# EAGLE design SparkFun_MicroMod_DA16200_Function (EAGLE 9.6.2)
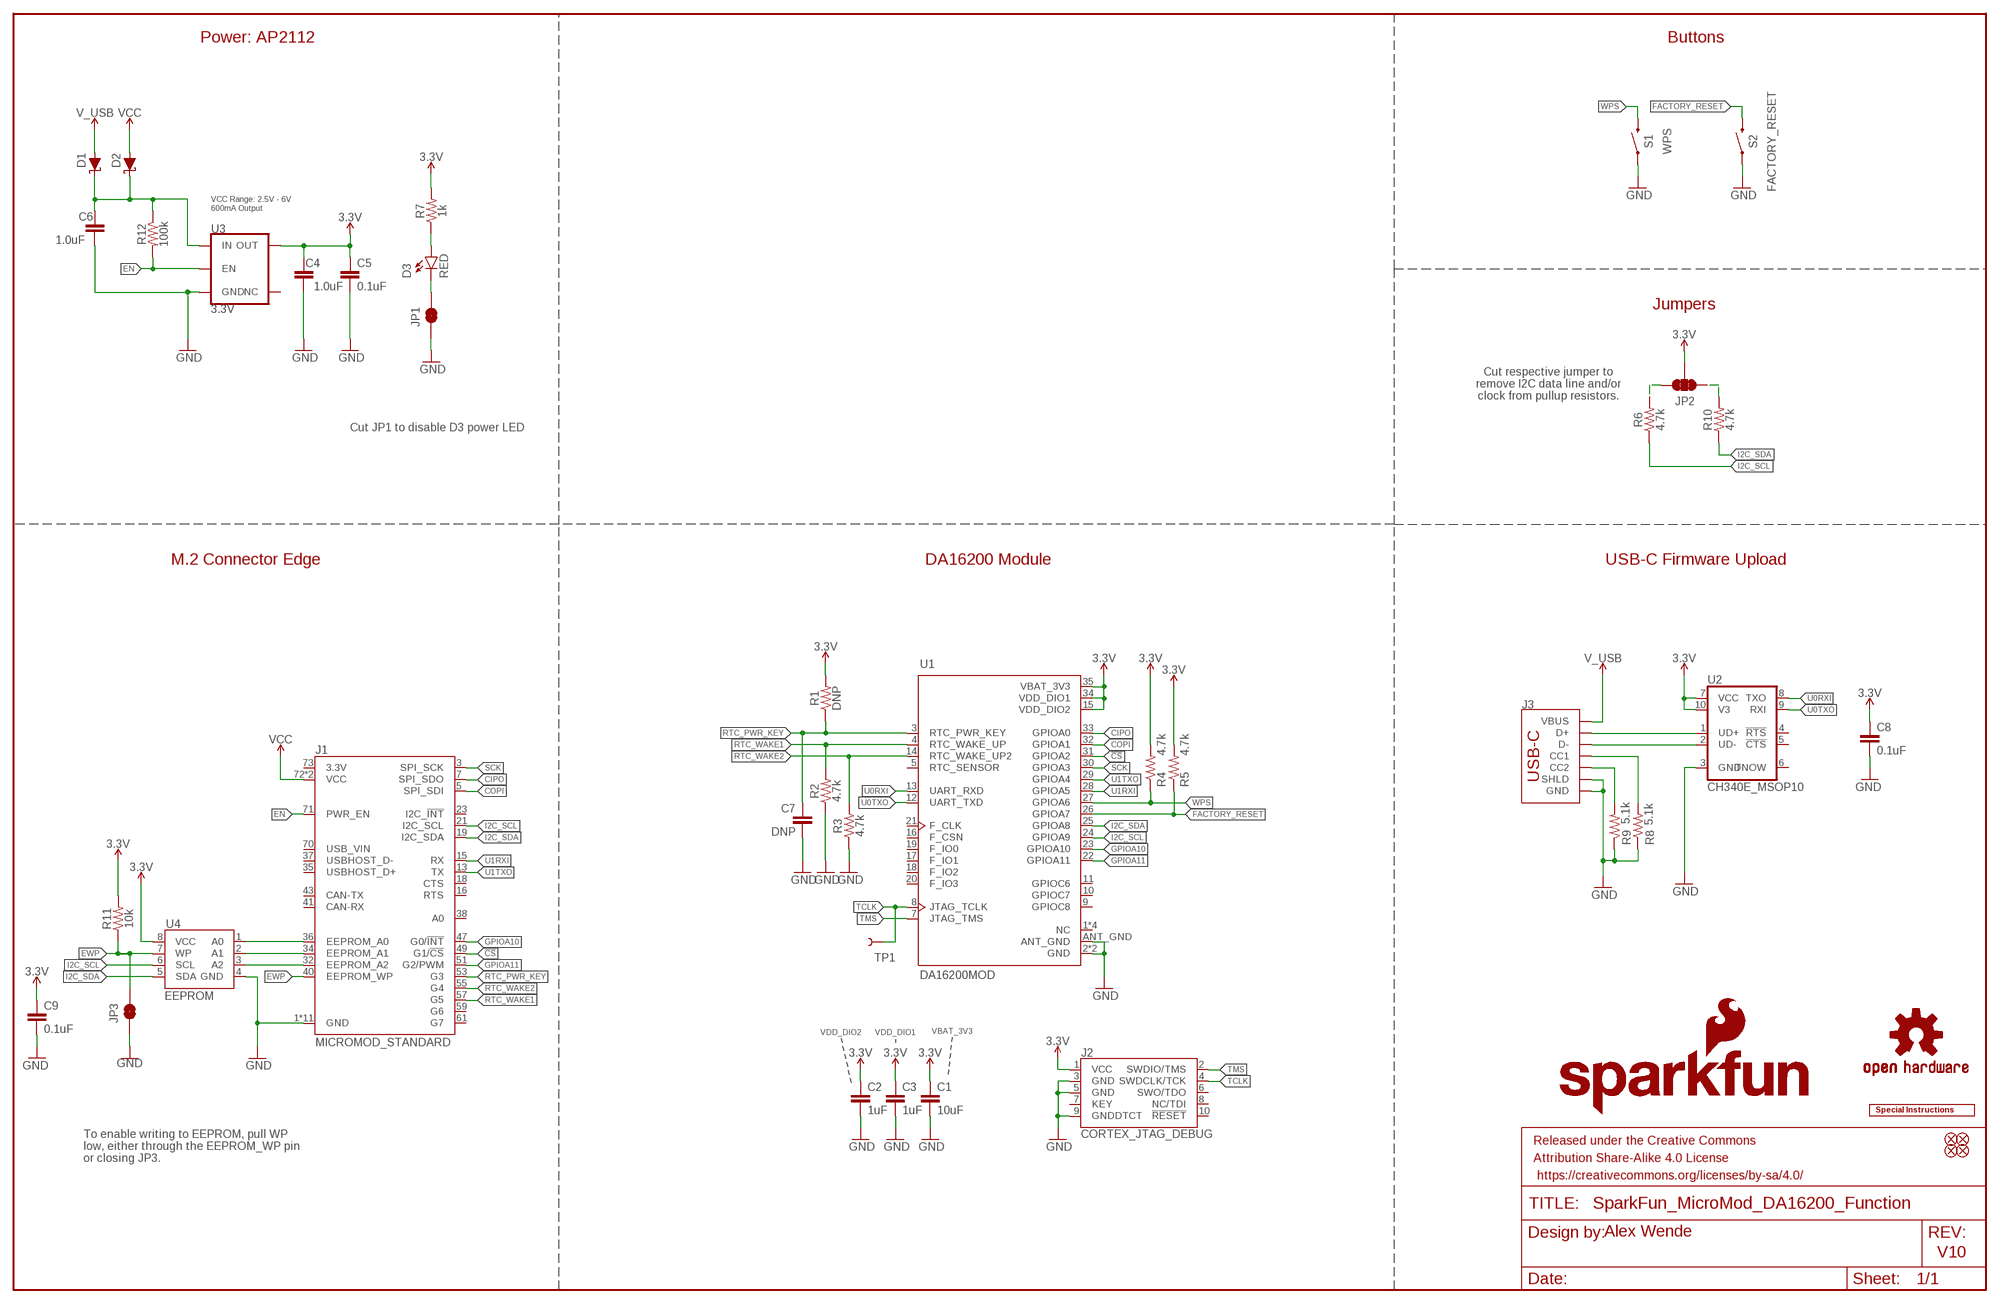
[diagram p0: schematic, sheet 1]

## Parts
C1  10uF  10UF-0603-6.3V-20%  [0603]
C2  1uF  1.0UF-0603-16V-10%  [0603]
C3  1uF  1.0UF-0603-16V-10%  [0603]
C4  1.0uF  1.0UF-0603-16V-10%  [0603]
C5  0.1uF  0.1UF-0603-25V-(+80/-20%)  [0603]
C6  1.0uF  1.0UF-0603-16V-10%  [0603]
C7  DNP  CAP-0603  [0603]
C8  0.1uF  0.1UF-0603-25V-(+80/-20%)  [0603]
C9  0.1uF  0.1UF-0603-25V-(+80/-20%)  [0603]
D1  DIODE-SCHOTTKY-BAT60A  [SOD-323]
D2  DIODE-SCHOTTKY-BAT60A  [SOD-323]
D3  RED  LED-0603_RIGHT_ANGLE  [LED-0603]
FD1  FIDUCIAL1X2  [FIDUCIAL-1X2]
FD2  FIDUCIAL1X2  [FIDUCIAL-1X2]
FD3  FIDUCIAL1X2  [FIDUCIAL-1X2]
FD4  FIDUCIAL1X2  [FIDUCIAL-1X2]
FRAME2  FRAME-LEDGER  [CREATIVE_COMMONS]
J1  MICROMOD_STANDARD  [M.2-CARD-E-22_FUNCTION_STANDARD]
J2  CORTEX_JTAG_DEBUG  CORTEX_JTAG_DEBUG_PTH_NS  [2X5-PTH-1.27MM-NO_SILK]
J3  USB_C_2-LAYER_PADS  [USB-C-16P-2LAYER-PADS]
JP1  JUMPER-SMT_2_NC_TRACE_SILK  [SMT-JUMPER_2_NC_TRACE_SILK]
JP2  JUMPER-SMT_3_2-NC_TRACE_SILK  [SMT-JUMPER_3_2-NC_TRACE_SILK]
JP3  JUMPER-SMT_2_NO_SILK  [SMT-JUMPER_2_NO_SILK]
LOGO1  SFE_LOGO_NAME_FLAME.2_INCH  [SFE_LOGO_NAME_FLAME_.2]
LOGO2  OSHW-LOGOS  [OSHW-LOGO-S]
LOGO3  SPECIAL_INSTRUCTIONS-ORDERING  [ORDERING_INSTRUCTIONS]
R1  DNP  RESISTOR0603  [0603]
R2  4.7k  4.7KOHM-0603-1/10W-1%  [0603]
R3  4.7k  4.7KOHM-0603-1/10W-1%  [0603]
R4  4.7k  4.7KOHM-0603-1/10W-1%  [0603]
R5  4.7k  4.7KOHM-0603-1/10W-1%  [0603]
R6  4.7k  4.7KOHM-0603-1/10W-1%  [0603]
R7  1k  1KOHM-0402T-1/16W-1%  [0402-TIGHT]
R8  5.1k  5.1KOHM-0402T-1/16W-1%  [0402-TIGHT]
R9  5.1k  5.1KOHM-0402T-1/16W-1%  [0402-TIGHT]
R10  4.7k  4.7KOHM-0603-1/10W-1%  [0603]
R11  10k  10KOHM-0603-1/10W-1%  [0603]
R12  100k  100KOHM-0603-1/10W-1%  [0603]
S1  WPS  MOMENTARY-SWITCH-SPST-SMD-5.2MM-TALL  [TACTILE_SWITCH_SMD_5.2MM]
S2  FACTORY_RESET  MOMENTARY-SWITCH-SPST-SMD-5.2MM-TALL  [TACTILE_SWITCH_SMD_5.2MM]
TP1  TEST-POINT3  [PAD.03X.03]
U1  DA16200MOD  DA16200MOD-AAC4WA32  [XCVR_DA16200MOD-AAC4WA32]
U2  CH340E_MSOP10  [MSOP10]
U3  3.3V  V_REG_AP2112K-3.3V  [SOT23-5]
U4  EEPROM  EEPROM-I2C512K  [SO08]

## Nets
3.3V: C1.1 C2.1 C3.1 C4.1 C5.1 C8.1 C9.1 J2.1(VCC) JP2.2 R1.2 R4.2 R5.2 R7.2 R11.2 U1.15(VDD_DIO2) U1.34(VDD_DIO1) U1.35(VBAT_3V3) U2.7(VCC) U2.10(V3) U3.5(OUT) U4.8(VCC)
!CS!: J1.49(G1/!CS!) U1.31(GPIOA2)
CIPO: J1.7(SPI_SDO) U1.33(GPIOA0)
COPI: J1.5(SPI_SDI) U1.32(GPIOA1)
EN: J1.71(PWR_EN) R12.2 U3.3(EN)
EWP: J1.40(EEPROM_WP) JP3.2 R11.1 U4.7(WP)
FACTORY_RESET: R5.1 S2.3 U1.26(GPIOA7)
GND: C1.2 C2.2 C3.2 C4.2 C5.2 C6.2 C7.2 C8.2 C9.2 J1.1(GND) J1.33(GND) J1.39(GND) J1.45(GND) J1.75(GND) J1.GND1(GND) J1.GND2(GND) J1.GND3(GND) J1.GND4(GND) J1.GND5(GND) J1.GND6(GND) J2.3(GND) J2.5(GND) J2.9(GNDDTCT) J3.GND J3.GND2(GND) J3.SHLD1(SHLD) J3.SHLD2(SHLD) J3.SHLD3(SHLD) J3.SHLD4(SHLD) JP1.1 JP3.1 R2.1 R3.1 R8.1 R9.1 S1.1 S2.1 U1.2(GND) U1.ANT_GND U1.GND U2.3(GND) U3.2(GND) U4.4(GND)
GPIOA10: J1.47(G0/!INT!) U1.23(GPIOA10)
GPIOA11: J1.51(G2/PWM) U1.22(GPIOA11)
I2C_SCL: J1.21(I2C_SCL) R6.1 U1.24(GPIOA9) U4.6(SCL)
I2C_SDA: J1.19(I2C_SDA) R10.1 U1.25(GPIOA8) U4.5(SDA)
N$1: J1.36(EEPROM_A0) U4.1(A0)
N$2: J3.A5(CC1) R8.2
N$3: C6.1 D1.C D2.C R12.1 U3.1(IN)
N$5: J3.B5(CC2) R9.2
N$6: D3.C JP1.2
N$7: D3.A R7.1
N$8: J1.32(EEPROM_A2) U4.3(A2)
N$9: J1.34(EEPROM_A1) U4.2(A1)
N$10: J3.A6(D+) J3.B6(D+) U2.1(UD+)
N$11: J3.A7(D-) J3.B7(D-) U2.2(UD-)
N$13: JP2.1 R10.2
N$14: JP2.3 R6.2
RTC_PWR_KEY: C7.1 J1.53(G3) R1.1 U1.3(RTC_PWR_KEY)
RTC_WAKE1: J1.57(G5) R2.2 U1.4(RTC_WAKE_UP)
RTC_WAKE2: J1.55(G4) R3.2 U1.14(RTC_WAKE_UP2)
SCK: J1.3(SPI_SCK) U1.30(GPIOA3)
TCLK: J2.4(SWDCLK/TCK) TP1.1 U1.8(JTAG_TCLK)
TMS: J2.2(SWDIO/TMS) U1.7(JTAG_TMS)
U0RXI: U1.13(UART_RXD) U2.8(TXO)
U0TXO: U1.12(UART_TXD) U2.9(RXI)
U1RXI: J1.15(RX) U1.28(GPIOA5)
U1TXO: J1.13(TX) U1.29(GPIOA4)
V_USB: D1.A J3.VBUS1(VBUS) J3.VBUS2(VBUS)
VCC: D2.A J1.72(VCC) J1.74(VCC)
WPS: R4.1 S1.3 U1.27(GPIOA6)
Unconnected: J1.16(RTS) J1.18(CTS) J1.23(I2C_!INT!) J1.35(USBHOST_D+) J1.37(USBHOST_D-) J1.38(A0) J1.41(CAN-RX) J1.43(CAN-TX) J1.59(G6) J1.61(G7) J1.70(USB_VIN) J1.73(3.3V) J2.6(SWO/TDO) J2.7(KEY) J2.8(NC/TDI) J2.10(!RESET) U1.1(NC) U1.5(RTC_SENSOR) U1.6(NC) U1.9(GPIOC8) U1.10(GPIOC7) U1.11(GPIOC6) U1.16(F_CSN) U1.17(F_IO1) U1.18(F_IO2) U1.19(F_IO0) U1.20(F_IO3) U1.21(F_CLK) U1.36(NC) U1.37(NC) U2.4(!RTS) U2.5(!CTS) U2.6(TNOW) U3.4(NC)

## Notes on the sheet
- Power: AP2112 | Buttons
- VCC Range: 2.5V - 6V 
  600mA Output
- Jumpers
- Cut respective jumper to
  remove I2C data line and/or
  clock from pullup resistors.
- Cut JP1 to disable D3 power LED
- M.2 Connector Edge | DA16200 Module | USB-C Firmware Upload
- VDD_DIO2 | VDD_DIO1 | VBAT_3V3
- To enable writing to EEPROM, pull WP
  low, either through the EEPROM_WP pin
  or closing JP3.
- Alex Wende
- V10

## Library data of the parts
C1 = SparkFun-Capacitors:10UF: 10.0µF ceramic capacitors; PROD_ID: CAP-11015
C2 C3 = SparkFun-Capacitors:1.0UF: 1µF ceramic capacitors; PROD_ID: CAP-00868; VALUE: 1.0uF
C4 C6 = SparkFun-Capacitors:1.0UF: 1µF ceramic capacitors; PROD_ID: CAP-00868
C5 C8 C9 = SparkFun-Capacitors:0.1UF: 0.1µF ceramic capacitors; PROD_ID: CAP-00810
C7 = SparkFun-Capacitors:CAP
D1 D2 = SparkFun-DiscreteSemi:DIODE-SCHOTTKY: Schottky diode; PROD_ID: DIO-14072; VALUE: 3A/10V/280mV
D3 = SparkFun-MicroMod-Function:LED-0603_RIGHT_ANGLE
FD1-FD4 = SparkFun-Aesthetics:FIDUCIAL: Fiducial Alignment Points
FRAME2 = SparkFun-Aesthetics:FRAME-LEDGER: Schematic Frame - Ledger
J1 = SparkFun-MicroMod-Function:MICROMOD: MicroMod Connector Description: A card edge connector and mating PCB connector to allow various MicroMod Processor Boards to be coupled with various carrier boards of different capabilities. Based on the M.2 standard.
J2 = SparkFun-Connectors:CORTEX_JTAG_DEBUG: Cortex Debug Connector - 10 pin Supports JTAG debug, Serial Wire debug, and Serial Wire Viewer. PTH and SMD connector options available. General Connector Information Products: PTH Connector -via Digi-Key SparkFun PSoc SparkFun T
J3 = SparkFun-Connectors:USB_C: USB Type C 16Pin Connector Super Speed pins not available on the 16-pin purely SMD connector so this part is best for USB 2.0 implementations. D1 and D2 are tied together enabling D+/- no matter which way the cable is plugged into the connector. The two channel configuration pins (CC1/2) are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; PROD_ID: CONN-14122
JP1 = SparkFun-Jumpers:JUMPER-SMT_2_NC_TRACE: Normally closed trace jumper
JP2 = SparkFun-Jumpers:JUMPER-SMT_3_2-NC_TRACE: Normally closed trace jumper (2 of 2 connections) This jumper has a trace between all three pads so they are normally closed (NC). Use a razor knife to open the connection(s). For best results follow the IPC guidelines for cutting traces: Cutout at least 0.063 mm (0.005 in). Remove all loose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
JP3 = SparkFun-Jumpers:JUMPER-SMT_2_NO: Normally open jumper
LOGO1 = SparkFun-Aesthetics:SFE_LOGO_NAME_FLAME: SparkFun Font Logo w/ Flame
LOGO2 = SparkFun-Aesthetics:OSHW-LOGO: Open-Source Hardware (OSHW) Logo
LOGO3 = SparkFun-Aesthetics:SPECIAL_INSTRUCTIONS: Special Ordering/Production Instructions Alert
R1 = SparkFun-Resistors:RESISTOR: Generic Resistor Package
R2-R6 R10 = SparkFun-Resistors:4.7KOHM: 4.7kΩ resistor; PROD_ID: RES-07857
R7 = SparkFun-Resistors:1KOHM: 1kΩ resistor; PROD_ID: RES-14342
R8 R9 = SparkFun-Resistors:5.1KOHM; PROD_ID: RES-14340
R11 = SparkFun-Resistors:10KOHM: 10kΩ resistor; PROD_ID: RES-00824
R12 = SparkFun-Resistors:100KOHM: 100kΩ resistor; PROD_ID: RES-07828
S1 S2 = SparkFun-Switches:MOMENTARY-SWITCH-SPST: Momentary Switch (Pushbutton) - SPST; PROD_ID: SWCH-14139
TP1 = SparkFun-Connectors:TEST-POINT: SparkFun Test Points
U1 = DA16200MOD:DA16200MOD-AAC4WA32: Check prices; PROD_ID: IC-16179
U2 = SparkFun-IC-Comms:CH340E; PROD_ID: IC-14135
U3 = SparkFun-IC-Power:V_REG_AP2112: AP2112 - 600mA CMOS LDO Regulator w/ Enable The AP2112 is CMOS process low dropout linear regulator with enable function, the regulator delivers a guaranteed 600mA (min.) continuous load current. Features Output Voltage Accuracy: ±1.5% Output Current: 600mA (Min.) Foldback Short Current Protection: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; PROD_ID: VREG-12457
U4 = SparkFun-IC-Memory:EEPROM-I2C: I2C EEPROMs, 24LC256 and others 24LC256 Series 256 kb I2C 2 Wire (32 k x 8 Bit) 2.5 V Serial EEPROM SMD - SOIC-8 Datasheet SparkFun Products SparkFun UDB5 - PIC UAV Development Board (GPS-11703); PROD_ID: IC-14645

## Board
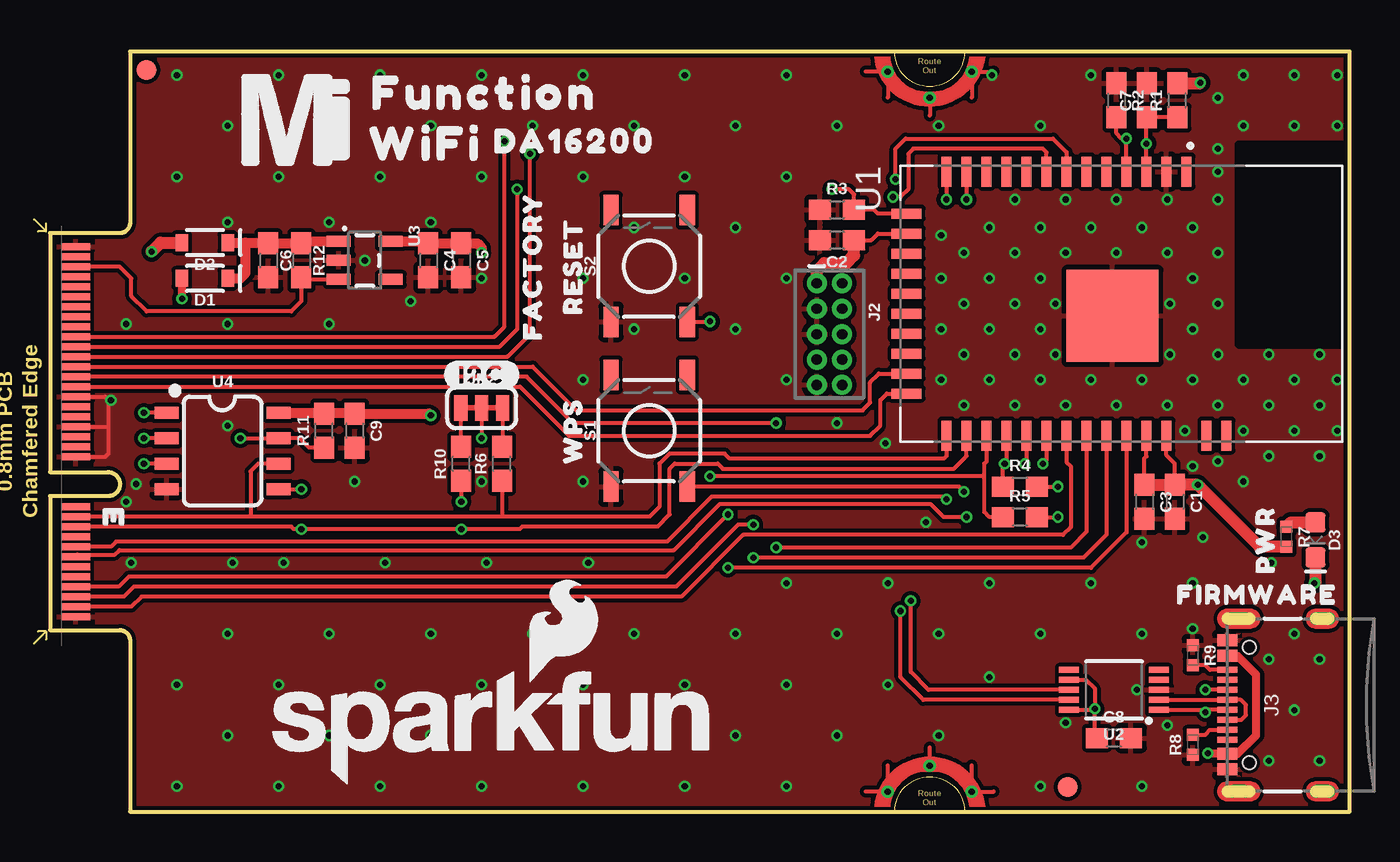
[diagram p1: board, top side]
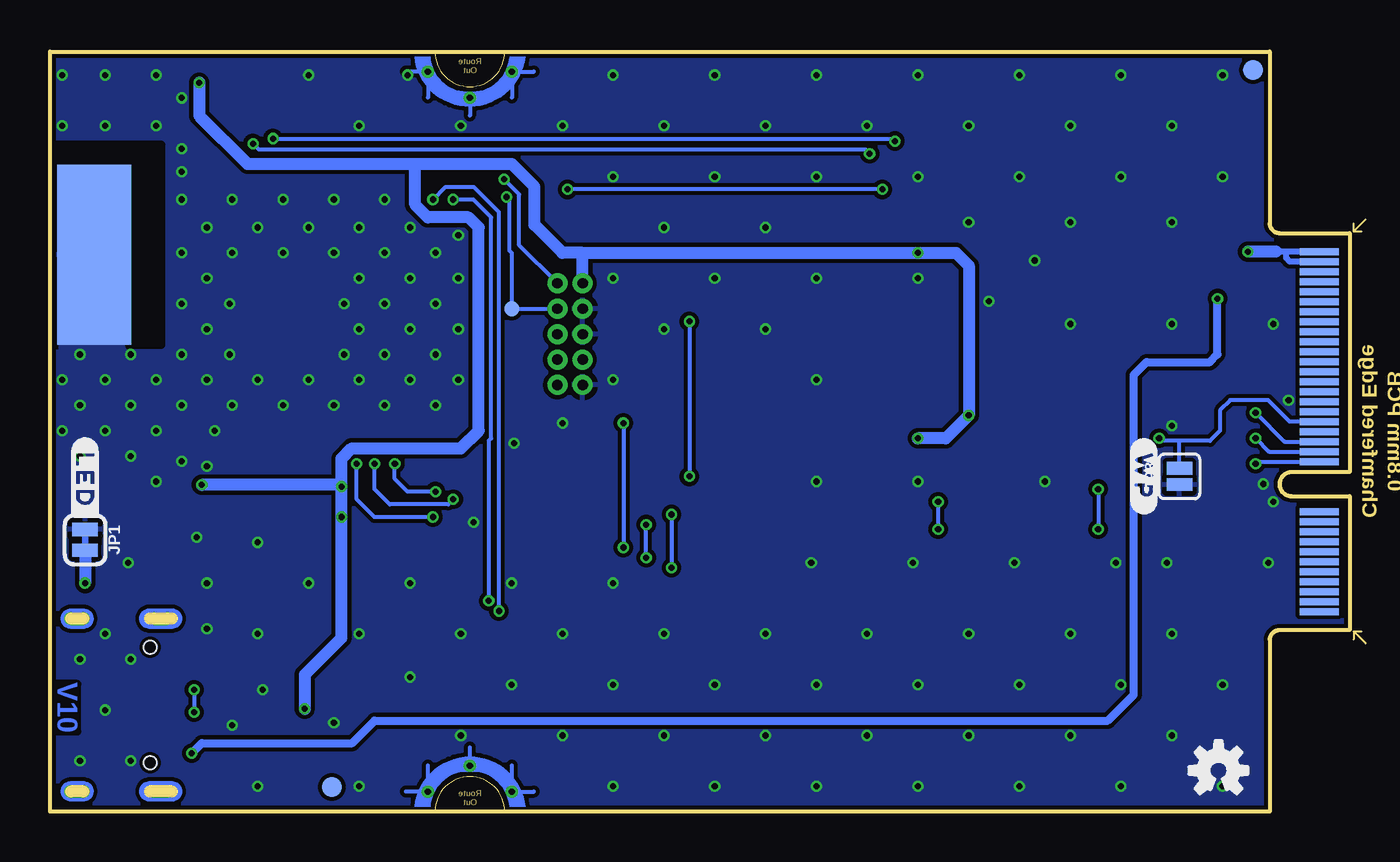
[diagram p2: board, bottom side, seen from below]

Size 65 x 38 mm. Coordinates in mm from the lower left corner, seen from the top.
Outline: 4,0 65,0 65,38 4,38 4,29.4 arc-84 3.5,28.93 0,28.93 0,16.98 2.9,16.98 arc-180 2.9,15.78 0,15.78 0,9.07 3.5,9.07 arc-85 4,8.6 4,0
Copper layers (1*16): Top 0.035mm / dielectric 1.5mm / Bottom 0.035mm
Design rules "SparkFun-2-Layer-Minimum-JLCPCB": minimum track width 5mil, minimum drill 0.3mm, track to track 5mil, track to pad 5mil, pad to pad 5mil, via to via 5mil, smd to smd 5mil, copper to edge 7mil, drill to drill 7mil, minimum pad ring 5mil, minimum via ring 5mil, stop-mask expansion 2.5mil, vias tented up to drill 25mil, thermal gap 10mil

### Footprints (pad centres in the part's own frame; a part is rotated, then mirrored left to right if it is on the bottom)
0603 = smd 1.1 x 1: 1 -0.85,0; 2 0.85,0
SOD-323 = smd 0.63 x 0.83: A 1.15,0; C -1.15,0
LED-0603 = smd 1 x 1: A -0.877,0; C 0.877,0
FIDUCIAL-1X2 = smd 1 x 1: 1 0,0
M.2-CARD-E-22_FUNCTION_STANDARD = smd 0.35 x 1.45: 1 9.25,1.275; 3 8.75,1.275; 5 8.25,1.275; 7 7.75,1.275; 9 7.25,1.275; 11 6.75,1.275; 13 6.25,1.275; 15 5.75,1.275; 17 5.25,1.275; 19 4.75,1.275; 21 4.25,1.275; 23 3.75,1.275; 33 1.25,1.275; 35 0.75,1.275; 37 0.25,1.275; 39 -0.25,1.275; 41 -0.75,1.275; 43 -1.25,1.275; 45 -1.75,1.275; 47 -2.25,1.275; 49 -2.75,1.275; 51 -3.25,1.275; 53 -3.75,1.275; 55 -4.25,1.275; 57 -4.75,1.275; 59 -5.25,1.275; 61 -5.75,1.275; 63 -6.25,1.275; 65 -6.75,1.275; 67 -7.25,1.275; 69 -7.75,1.275; 71 -8.25,1.275; 73 -8.75,1.275; 75 -9.25,1.275 | smd 0.35 x 1.95 bottom: 2 9,1.525; 4 8.5,1.525; 6 8,1.525; 8 7.5,1.525; 10 7,1.525; 12 6.5,1.525; 14 6,1.525; 16 5.5,1.525; 18 5,1.525; 20 4.5,1.525; 22 4,1.525; 32 1.5,1.525; 34 1,1.525; 36 0.5,1.525; 38 0,1.525; 40 -0.5,1.525; 42 -1,1.525; 44 -1.5,1.525; 46 -2,1.525; 48 -2.5,1.525; 50 -3,1.525; 52 -3.5,1.525; 54 -4,1.525; 56 -4.5,1.525; 58 -5,1.525; 60 -5.5,1.525; 62 -6,1.525; 64 -6.5,1.525; 66 -7,1.525; 68 -7.5,1.525; 70 -8,1.525; 72 -8.5,1.525; 74 -9,1.525 | drill 0.305 pad 0.61: GND1 -18,41.9; GND2 -16.7,44; GND3 -18,46.1; GND4 18,41.9; GND5 16.7,44; GND6 18,46.1
2X5-PTH-1.27MM-NO_SILK = drill 0.508 pad 1: 1 -2.54,-0.635; 2 -2.54,0.635; 3 -1.27,-0.635; 4 -1.27,0.635; 5 0,-0.635; 6 0,0.635; 7 1.27,-0.635; 8 1.27,0.635; 9 2.54,-0.635; 10 2.54,0.635
USB-C-16P-2LAYER-PADS = smd 0.3 x 1: A5 -1.25,-0.34; A6 -0.25,-0.34; A7 0.25,-0.34; A8 1.25,-0.34; B5 1.75,-0.34; B6 0.75,-0.34; B7 -0.75,-0.34; B8 -1.75,-0.34 | smd 0.6 x 1: GND -3.225,-0.34; GND2 3.225,-0.34; VBUS1 -2.45,-0.34; VBUS2 2.45,-0.34 | drill 0.4 pad 0.6 long: SHLD1 -4.318,-0.915; SHLD2 4.318,-0.915; SHLD3 -4.318,-5.095; SHLD4 4.318,-5.095 | hole 0.65: -2.89,-1.445; 2.89,-1.445
SMT-JUMPER_2_NC_TRACE_SILK = smd 0.66 x 1.27: 1 -0.521,0; 2 0.521,0
SMT-JUMPER_3_2-NC_TRACE_SILK = smd 0.66 x 1.27: 1 -1.041,0; 2 0,0; 3 1.041,0
SMT-JUMPER_2_NO_SILK = smd 0.635 x 1.27: 1 -0.406,0; 2 0.406,0
0402-TIGHT = smd 0.6 x 0.6: 1 -0.5,0; 2 0.5,0
TACTILE_SWITCH_SMD_5.2MM = smd 1.524 x 0.762: 1 -2.794,1.905; 2 2.794,1.905; 3 -2.794,-1.905; 4 2.794,-1.905
PAD.03X.03 = smd 0.762 x 0.762: 1 0,0
XCVR_DA16200MOD-AAC4WA32 = smd 1.5 x 0.5: 1 -6.6,3.25; 2 -6.6,2.25; 3 -6.6,1.25; 4 -6.6,0.25; 5 -6.6,-0.75; 6 -6.6,-1.75; 7 -6.6,-2.75; 8 -6.6,-3.75; 9 -6.6,-4.75; 10 -6.6,-5.75; 11 -6.6,-6.75; 12 -6.6,-7.75; 13 -6.6,-8.75; 24 6.6,-8.75; 25 6.6,-7.75; 26 6.6,-6.75; 27 6.6,-5.75; 28 6.6,-4.75; 29 6.6,-3.75; 30 6.6,-2.75; 31 6.6,-1.75; 32 6.6,-0.75; 33 6.6,0.25; 34 6.6,1.25; 35 6.6,2.25; 36 6.6,4.25; 37 6.6,5.25 | smd 0.5 x 1.5: 14 -4.5,-10.75; 15 -3.5,-10.75; 16 -2.5,-10.75; 17 -1.5,-10.75; 18 -0.5,-10.75; 19 0.5,-10.75; 20 1.5,-10.75; 21 2.5,-10.75; 22 3.5,-10.75; 23 4.5,-10.75 | smd 9 x 3.7 bottom: ANT_GND -2.45,9.2 | smd 4.6 x 4.6: GND 0.61,-0.45
MSOP10 = smd 1 x 0.3: 1 -2.25,1; 2 -2.25,0.5; 3 -2.25,0; 4 -2.25,-0.5; 5 -2.25,-1; 6 2.25,-1; 7 2.25,-0.5; 8 2.25,0; 9 2.25,0.5; 10 2.25,1
SOT23-5 = smd 0.55 x 1.2: 1 -0.95,-1.3; 2 0,-1.3; 3 0.95,-1.3; 4 0.95,1.3; 5 -0.95,1.3
SO08 = smd 0.6 x 1.2: 1 -1.905,-2.8; 2 -0.635,-2.8; 3 0.635,-2.8; 4 1.905,-2.8; 5 1.905,2.8; 6 0.635,2.8; 7 -0.635,2.8; 8 -1.905,2.8

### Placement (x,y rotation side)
C1  56.26,15.49 270 top
C2  39.37,28.57 180 top
C3  54.74,15.49 270 top
C4  18.92,27.56 270 top
C5  20.57,27.56 270 top
C6  10.92,27.56 270 top
C7  54.86,35.56 90 top
C8  53.21,3.68 0 top
C9  15.24,19.05 270 top
D1  7.75,26.67 180 top
D2  7.75,28.45 180 top
D3  63.3,13.59 270 top
FD1  4.83,37.08 0 top
FD2  4.83,37.08 0 bottom
FD3  50.9,1.24 0 top
FD4  50.9,1.24 0 bottom
FRAME2  not placed on the board
J1  0,19 270 top
J2  38.99,23.88 270 top
J3  58.55,5.33 90 top
JP1  63.25,13.59 270 bottom
JP2  21.59,20.19 0 top
JP3  8.51,16.76 90 bottom
LOGO1  22.12,4.22 0 top
LOGO2  6.55,2.06 0 bottom
LOGO3  not placed on the board
R1  56.39,35.56 90 top
R2  53.34,35.56 270 top
R3  39.37,30.1 0 top
R4  48.51,16.26 0 top
R5  48.51,14.73 0 top
R6  22.61,17.4 90 top
R7  61.85,13.74 270 top
R8  57.15,3.34 90 top
R9  57.15,7.82 270 top
R10  20.57,17.4 90 top
R11  13.72,19.05 90 top
R12  12.57,27.56 270 top
S1  29.97,19.05 90 top
S2  29.97,27.28 90 top
TP1  41.91,25.15 0 bottom
U1  53.59,25.4 270 top
U2  53.21,6.1 180 top
U3  15.75,27.56 270 top
U4  8.64,18.03 270 top
U$1  [FIRMWARE0]  60.38,10.85 0 top
U$2  [PWR0]  60.78,13.59 90 top
U$3  [#LED#0]  63.25,14.48 270 bottom
U$4  [FUNCTION0]  21.72,35.94 0 top
U$5  [DA162000]  26.24,33.53 0 top
U$6  [WIFI0]  18.8,33.4 0 top
U$7  [WPS0]  26.16,19.05 90 top
U$8  [FACTORY0]  24.13,27.28 90 top
U$9  [RESET0]  26.16,27.28 90 top
U$10  [#WP#0]  10.29,16.76 270 bottom
U$11  [#I2C#0]  21.59,21.84 0 top
U$12  [MICROMOD_MI_LOGO_1]  12.32,34.62 0 top

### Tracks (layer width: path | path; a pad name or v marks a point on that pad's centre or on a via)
3.3V  (via drill 0.3)
  Top 0.203: R5.2 v50.42,14.73 | R4.2 v50.42,16.26 | C3.1 54.74,17.65 54.84,17.76 U1.34 | C1.1 56.26,17.4 55.84,17.82 U1.35 | C2.1 41.08,28.57 41.4,28.9 U1.15 | C8.1 52.26,3.79 v52.26,5.14 | U2.10 52.21,5.1 v52.26,5.14 | U2.7 51.82,6.6 52.26,6.16 v52.26,5.14 | JP2.2 v21.59,18.67
  Top 0.508: U3.5 18.82,28.51 C4.1 C5.1 21.38,28.41 21.59,28.19 v21.59,27.94 | U4.8 13.68,19.94 R11.2 13.76,19.94 15.24,19.94 C9.1 18.96,19.9 v19.05,19.81
  Top 0.61: R7.2 60.51,13.24 v57.4,16.34 C1.1 C3.1 | R1.2 57.49,36.41 v57.53,36.45 | J2.1 38.35,27.05 38.73,27.43 39.84,27.43 40.22,27.81 C2.1
  Bottom 0.61: v52.26,5.14 52.26,6.86 50.42,8.7 v50.42,14.73 v50.42,16.26 | v50.42,16.26 50.42,16.34 v57.4,16.34 | v57.53,36.45 57.53,34.8 55.12,32.38 46.74,32.38 | 46.74,32.38 41.91,32.38 40.77,31.24 40.77,29.34 39.37,27.94 38.35,27.94 | J2.1 38.35,27.94 | 38.35,27.94 v21.59,27.94 19.68,27.94 19.05,27.3 v19.05,19.81 20.19,18.67 v21.59,18.67 | 46.74,32.38 46.74,30.35 46.1,29.72 44.07,29.72 43.56,29.21 43.56,19.05 44.45,18.16 49.91,18.16 50.42,17.65 v50.42,16.26
!CS!  (via drill 0.3)
  Top 0.203: U1.31 51.84,14 51.05,13.21 v36.32,13.21 | v36.32,19.43 26.16,19.43 23.84,21.75 J1.49
  Bottom 0.203: v36.32,19.43 v36.32,13.21
CIPO  (via drill 0.3)
  Top 0.203: U1.33 53.84,13.97 52.07,12.19 v33.91,12.19 | v33.91,14.86 30.81,11.76 3.94,11.76 3.43,11.25 J1.7
  Bottom 0.203: v33.91,14.86 v33.91,12.19
COPI  (via drill 0.3)
  Top 0.203: U1.32 52.84,13.86 51.69,12.7 v35.18,12.7 | v35.18,14.35 34.42,14.35 31.32,11.26 4.2,11.26 3.69,10.75 J1.5
  Bottom 0.203: v35.18,12.7 v35.18,14.35
EN
  Top 0.203: J1.71 3.48,27.25 4.06,26.67 4.06,25.78 4.83,25.02 12.06,25.02 12.57,25.53 R12.2 12.67,26.61 U3.3
EWP  (via drill 0.3)
  Top 0.203: R11.1 12.95,18.2 12.48,18.67 U4.7 v9.53,18.67
  Bottom 0.203: J1.40 2.99,19.5 4.06,20.57 5.97,20.57 6.48,20.07 6.48,19.05 6.99,18.54 8.51,18.54 | 8.51,18.54 9.4,18.54 v9.53,18.67 | JP3.2 8.51,18.54
FACTORY_RESET  (via drill 0.3)
  Top 0.203: U1.26 46.84,17.51 46.74,17.4 46.74,16.76 | R5.1 46.99,14.73 46.74,14.99 46.74,16.76 | 46.74,16.76 v33.02,16.76 | S2.3 32.99,24.49 v33.02,24.51
  Bottom 0.203: v33.02,24.51 v33.02,16.76
GND  (via drill 0.3)
  Top 0.203: J1.GND4 42.67,1.77 42.67,2.03 42.94,2.3 J1.GND5 45.07,2.3 46.1,1.27 J1.GND6 | J1.GND1 41.9,36.59 42.16,36.32 42.67,36.32 43.29,35.7 J1.GND2 44.82,35.7 44.83,35.69 45.21,35.69 46.1,36.58 J1.GND3 | J1.33 2.76,17.75 2.92,17.91 2.92,19.25 | J1.45 2.75,20.75 2.92,20.57 2.92,19.25 | J1.39 2.92,19.25
  other vias: 55.88,30.61 58.42,30.61 53.34,30.61 50.8,30.61 48.26,30.61 57.15,29.21 54.61,29.21 52.07,29.21 49.53,29.21 46.99,29.21 58.42,27.94 55.88,27.94 53.34,27.94 50.8,27.94 48.26,27.94 45.72,27.94 44.58,28.83 46.99,26.67 46.99,24.13 46.99,21.59 48.26,25.4 48.26,22.86 48.26,20.32 45.72,20.32 45.72,22.86 45.72,25.4 49.53,26.67 49.53,24.13 49.53,21.59 50.8,20.32 53.34,20.32 55.88,20.32 58.42,20.32 60.96,20.32 63.5,20.32 52.07,21.59 54.61,21.59 57.15,21.59 59.69,21.59 62.23,21.59 64.39,21.59 63.5,22.86 60.96,22.86 58.42,22.86 58.42,25.4 58.42,33.15 58.42,35.69 59.69,34.29 62.23,34.29 64.39,34.29 59.69,36.83 62.23,36.83 64.39,36.83 58.42,32 52.07,36.83 49.53,34.29 47.12,36.83 44.45,34.29 57.15,24.13 57.15,26.67 56.01,25.4 56.01,22.86 50.29,25.4 50.29,22.86 3.81,24.38 3.81,15.49 64.39,19.05 62.23,19.05 59.69,19.05 56.77,19.05 59.69,16.51 63.5,17.78 60.96,17.78 58.42,17.53 57.15,17.27 57.15,11.43 52.07,11.43 61.09,12.45 57.66,13.72 54.61,13.46 57.15,9.14 62.23,8.89 62.23,5.08 63.5,2.54 63.5,7.62 60.96,7.62 60.96,2.54 54.61,1.27 49.53,1.27 50.8,4.45 44.45,3.81 39.37,3.81 34.29,3.81 29.21,3.81 24.13,3.81 19.05,3.81 13.97,3.81 8.89,3.81 6.35,1.27 11.43,1.27 16.51,1.27 21.59,1.27 26.67,1.27 31.75,1.27 36.83,1.27 41.91,6.35 36.83,6.35 31.75,6.35 26.67,6.35 21.59,6.35 16.51,6.35 11.43,6.35 6.35,6.35 46.99,6.73 46.99,11.43 54.36,6.1 55.88,4.32 44.58,21.59 44.58,24.13 44.58,26.67 43.81,14.48 4.06,12.45 6.35,31.75 6.35,36.83 8.89,8.89 8.89,19.3 8.89,24.38 8.89,29.46 8.89,34.29 11.43,31.75 11.43,36.83 13.97,8.89 13.97,24.38 13.97,29.46 13.97,34.29 15.75,27.56 16.51,31.75 16.51,36.83 19.05,8.89 18.03,25.53 19.05,29.46 19.05,34.29 21.59,16.51 21.59,26.67 21.59,31.75 21.59,36.83 24.13,8.89 41.91,11.43 39.37,8.89 39.37,19.43 36.83,11.43 36.83,21.59 36.83,26.67 36.83,31.75 34.29,8.89 34.29,24.13 34.29,29.21 29.21,8.89 29.21,24.13 29.21,29.21 26.67,16.51 26.67,21.59 26.67,26.67 26.67,31.75 31.75,26.67 31.75,31.75 34.29,34.29 39.37,34.29 24.13,34.29 29.21,34.29 26.67,36.83 31.75,36.83 36.83,36.83 15.24,16.51 44.45,8.89 49.53,8.89 54.61,8.89 3.05,20.57 4.32,16.38 9.14,12.45 11.68,12.45 16.76,12.45 21.84,12.45 26.92,12.45 41.78,18.41
  pour Top (isolate 0.203): 0,0 0,38 65,38 65,0
  pour Bottom (isolate 0.203): 0,38 0,0 65,0 65,38
  pour Bottom (isolate 0.305, no thermals): 60.75,24 64.51,24 64.51,22 60.75,22
GPIOA10
  Top 0.203: J1.47 23.5,21.25 25.95,18.8 41.02,18.8 41.53,19.3 41.53,20.57 41.85,20.9 U1.23
GPIOA11
  Top 0.203: J1.51 24.14,22.25 26.32,20.07 40.64,20.07 41.02,20.45 41.02,21.46 41.46,21.9 U1.22
I2C_SCL
  Top 0.203: U1.24 44.84,17.79 44.7,17.65 33.99,17.65 33.74,17.91 30.99,17.91 30.48,17.4 30.48,15.24 29.99,14.75 22.61,14.75 | 22.61,14.75 10.03,14.75 | 10.03,14.75 J1.21 | R6.1 22.61,14.75 | U4.6 10.41,17.4 10.03,17.02 10.03,14.75
I2C_SDA  (via drill 0.3)
  Top 0.203: U1.25 45.85,17.78 45.21,17.14 33.66,17.14 33.4,17.4 31.24,17.4 30.99,17.14 30.99,14.86 30.38,14.25 23.62,14.25 23.5,14.12 v20.57,14.12 v12.57,14.12 12.19,14.12 12.06,14.25 J1.19 | U4.5 v12.57,16.13 | R10.1 v20.57,15.49
  Bottom 0.203: v20.57,14.12 v20.57,15.49 | v12.57,16.13 v12.57,14.12
N$1  (via drill 0.3)
  Top 0.203: U4.1 v4.7,19.94
  Bottom 0.203: v4.7,19.94 3.26,18.5 J1.36
N$2
  Top 0.203: R8.2 57.78,3.85 58.02,4.08 J3.A5
N$3
  Top 0.508: D2.C 9.78,28.45 | 9.78,28.45 10.88,28.45 C6.1 R12.1 12.67,28.51 U3.1 | D1.C 9.53,26.67 9.78,26.92 9.78,28.45
N$5
  Top 0.203: J3.B5 58.02,7.08 57.78,7.32 R9.2
N$6  (via drill 0.3)
  Top 0.61: D3.C 63.3,11.48 v63.25,11.43
  Bottom 0.61: JP1.2 v63.25,11.43
N$7
  Top 0.61: R7.1 62.07,14.47 D3.A
N$8  (via drill 0.3)
  Top 0.203: U4.3 v4.7,17.4
  Bottom 0.203: v4.7,17.4 4.6,17.5 J1.32
N$9  (via drill 0.3)
  Top 0.203: U4.2 v4.7,18.67
  Bottom 0.203: v4.7,18.67 4.03,18 J1.34
N$10  (via drill 0.3)
  Top 0.203: J3.A6 57.87,5.08 57.78,5 v57.78,4.97 57.75,4.97 57.62,5.1 U2.1 | J3.B6 57.8,6.08 v57.78,6.1
  Bottom 0.203: v57.78,6.1 v57.78,4.97
N$11
  Top 0.203: U2.2 55.48,5.58 J3.A7 59.57,5.58 59.82,5.33 59.82,4.83 59.58,4.58 J3.B7
N$13
  Top 0.203: R10.2 20.55,18.27 JP2.1
N$14
  Top 0.203: JP2.3 22.63,18.27 R6.2
RTC_PWR_KEY  (via drill 0.3)
  Top 0.203: R1.1 C7.1 54.84,34.71 v54.84,33.4 U1.3 | J1.53 22.88,22.75 24,23.88 v24,32.89
  Bottom 0.203: v54.84,33.4 54.54,33.1 24.21,33.1 v24,32.89
RTC_WAKE1  (via drill 0.3)
  Top 0.203: U1.4 v53.84,33.66 53.59,33.66 53.34,33.91 R2.2 | J1.57 22.23,23.75 22.73,24.26 v22.73,33.53
  Bottom 0.203: v53.84,33.66 22.86,33.66 v22.73,33.53
RTC_WAKE2  (via drill 0.3)
  Top 0.203: J1.55 22.49,23.25 23.37,24.13 v23.37,31.11 | U1.14 41.4,29.9 41.2,30.1 R3.2 40.22,30.86 39.97,31.11 v39.12,31.11
  Bottom 0.203: v23.37,31.11 v39.12,31.11
SCK
  Top 0.203: U1.30 50.84,17.48 51.05,17.27 51.05,14.22 50.67,13.84 34.67,13.84 31.59,10.76 4.58,10.76 4.07,10.25 J1.3
TCLK  (via drill 0.3)
  Top 0.203: U1.8 49.84,32.96 49.66,33.15 43.18,33.15 42.93,32.89 42.93,31.11 42.55,30.73 v42.16,30.73
  Bottom 0.203: J2.4 TP1.1 41.91,27.94 42.04,28.07 42.04,30.61 v42.16,30.73
TMS  (via drill 0.3)
  Top 0.203: U1.7 50.84,32.98 50.16,33.66 42.8,33.66 42.29,33.15 v42.29,31.62
  Bottom 0.203: J2.2 41.53,28.32 41.53,30.86 v42.29,31.62
U0RXI  (via drill 0.3)
  Top 0.203: U1.13 44.84,30.61 v44.83,30.61 | U2.8 43.94,6.1 43.05,6.99 v43.05,10.54
  Bottom 0.203: v43.05,10.54 43.05,18.54 42.93,18.67 42.93,29.72 43.81,30.61 v44.83,30.61
U0TXO  (via drill 0.3)
  Top 0.203: U1.12 v45.84,30.61 v45.85,30.61 | U2.9 43.68,5.6 42.55,6.73 v42.55,10.03
  Bottom 0.203: v42.55,10.03 42.55,29.97 43.81,31.24 45.21,31.24 v45.85,30.61
U1RXI  (via drill 0.3)
  Top 0.203: U1.28 48.84,17.48 v48.77,17.4 | v44.83,15.62 44.7,15.75 33.1,15.75 30.85,13.5 3.31,13.5 3.05,13.25 J1.15
  Bottom 0.203: v44.83,15.62 45.09,15.37 48.01,15.37 48.77,16.13 v48.77,17.4
U1TXO  (via drill 0.3)
  Top 0.203: U1.29 49.84,17.59 v49.66,17.4 | v45.85,14.73 44.7,14.73 44.07,15.37 33.49,15.37 31.2,13.08 3.48,13.08 3.24,12.85 1.37,12.85 J1.13
  Bottom 0.203: v45.85,14.73 48.77,14.73 49.66,15.62 v49.66,17.4
V_USB  (via drill 0.3)
  Top 0.203: 6.6,25.66 v6.6,25.65
  Top 0.406: J3.VBUS2 59.4,7.78 60.33,6.86 60.33,3.81 59.4,2.88 J3.VBUS1 57.95,2.88 v57.91,2.92 | D1.A 6.6,25.66
  Bottom 0.406: v57.91,2.92 57.4,3.43 49.88,3.43 48.77,4.55 12.09,4.55 10.79,5.84 10.79,21.84 10.16,22.48 6.99,22.48 6.6,22.86 v6.6,25.65
VCC  (via drill 0.3)
  Top 0.61: v5.08,28 5.53,28.45 D2.A
  Bottom 0.305: J1.74 3.17,28 | 3.17,28 3.68,28 | J1.72 2.99,27.5 3.17,27.69 3.17,28
  Bottom 0.61: 3.68,28 v5.08,28
WPS  (via drill 0.3)
  Top 0.203: U1.27 47.84,17.49 v47.75,17.4 47.66,17.31 R4.1 | S1.3 45.47,16.26 v45.72,16
  Bottom 0.203: v45.72,16 47.12,16 47.75,16.64 v47.75,17.4

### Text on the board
Bottom: V10
tDocu: 0.8mm PCB / ENIG Finish / 45 degree chamfered edge | Alex Wende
